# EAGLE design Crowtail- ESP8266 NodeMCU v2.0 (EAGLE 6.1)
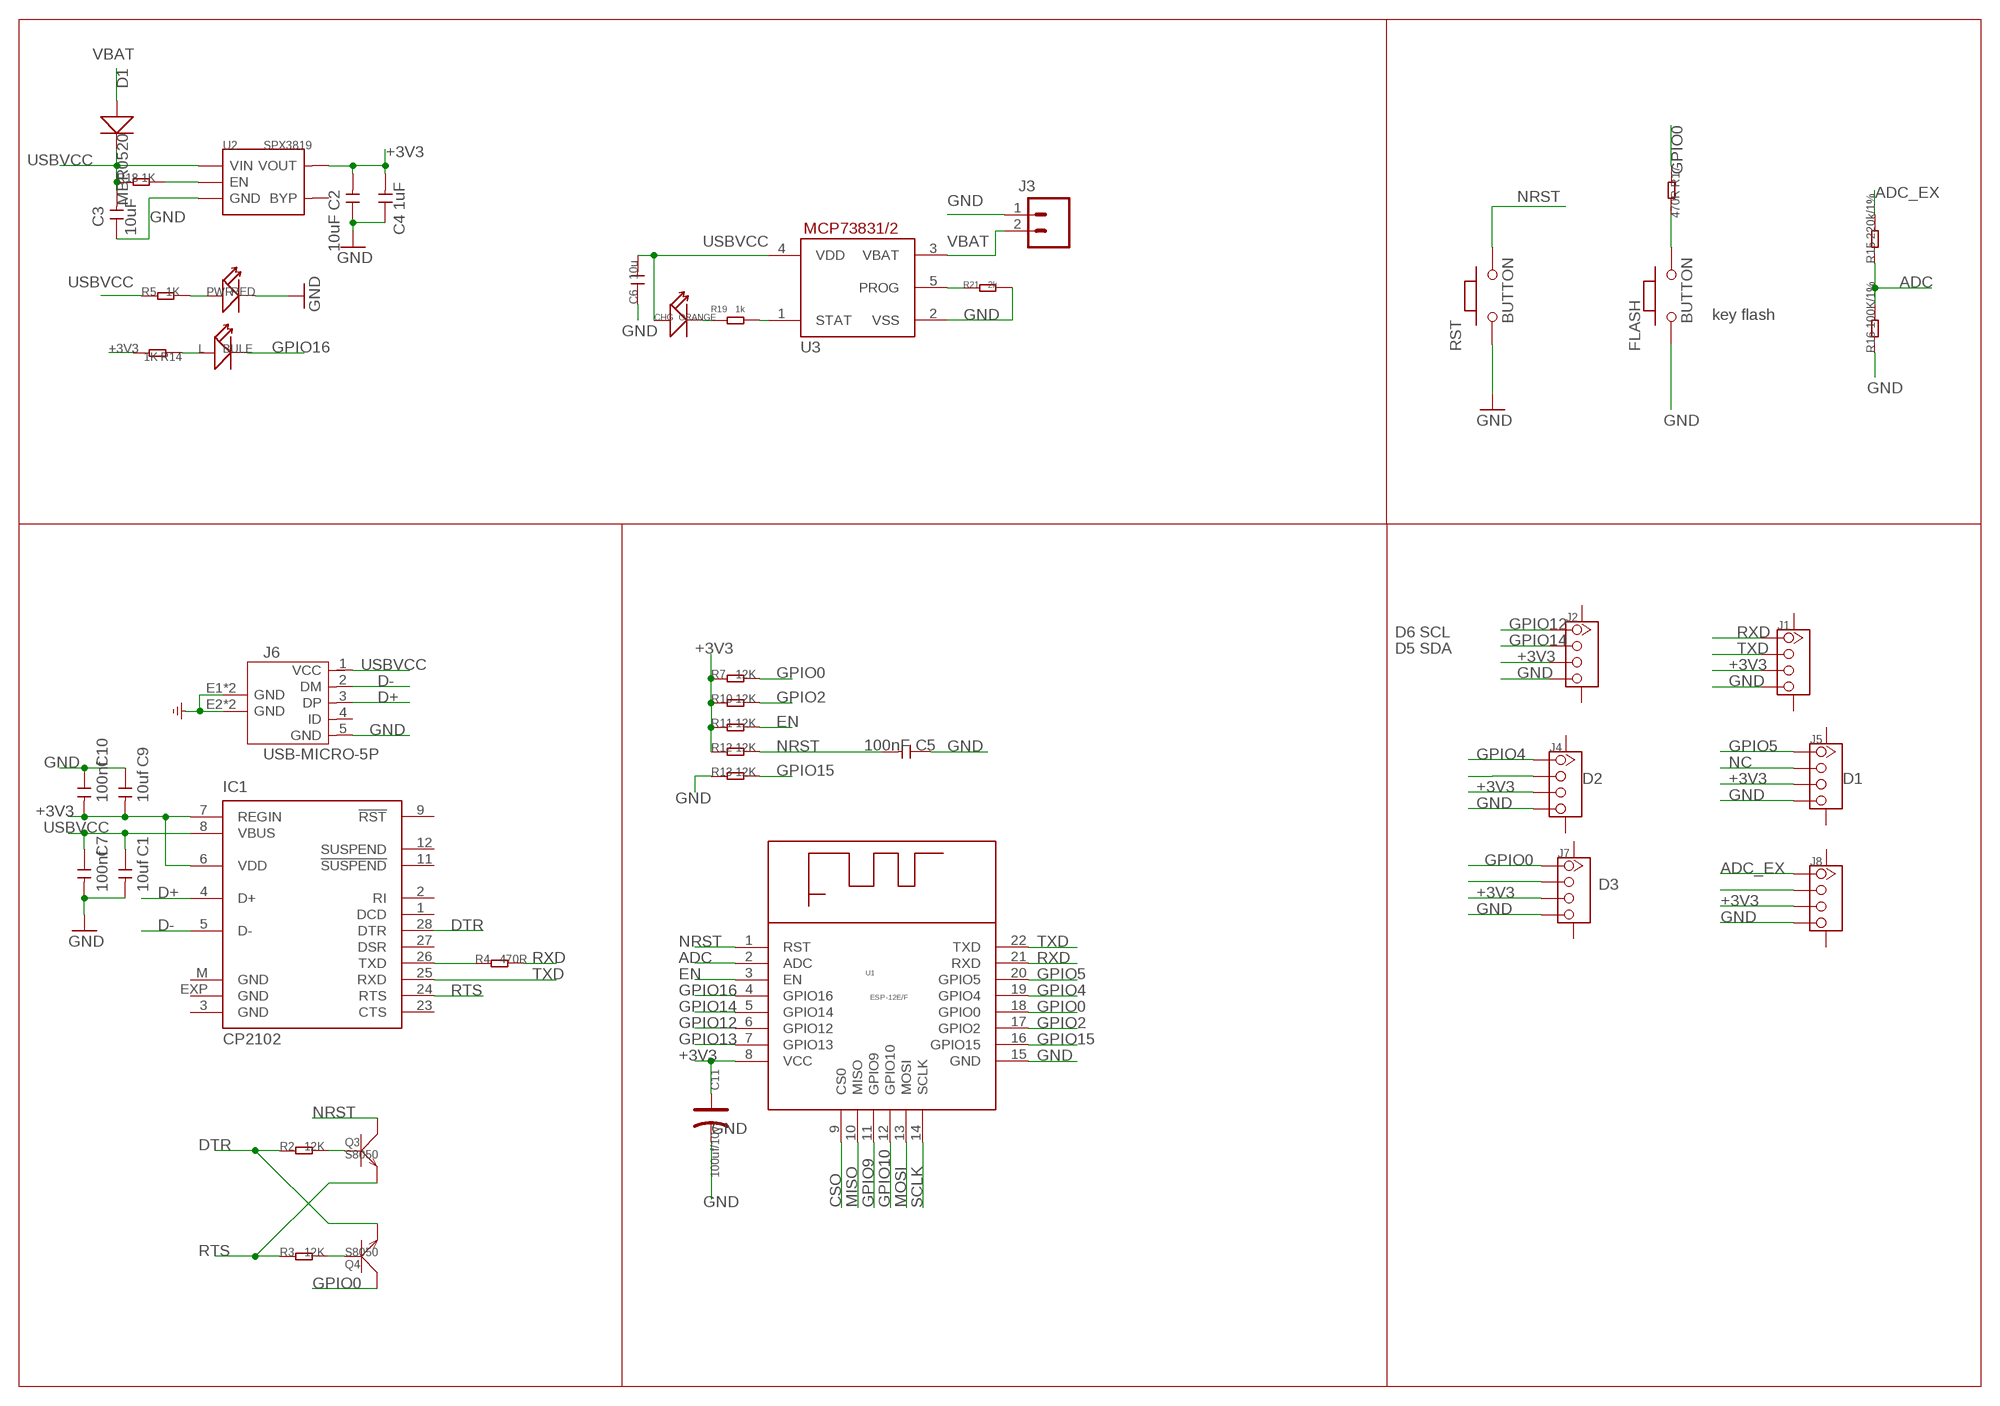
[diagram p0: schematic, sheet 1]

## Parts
C1  10uf  C-0603  [C0603]
C2  10uF  C-0603  [C0603]
C3  10uF  C-0603  [C0603]
C4  1uF  C-0603  [C0603]
C5  100nF  C-0603  [C0603]
C6  10u  C-0603  [C0603]
C7  100nf  C-0603  [C0603]
C9  10uf  C-0603  [C0603]
C10  100nf  C-0603  [C0603]
C11  100uf/10v  CAP-AVX-B  [AVX-B]
CHG  ORANGE  007-LED0603  [D0603]
D1  MBR0520  D'1206'  [SOD123]
FLASH  BUTTON  PB157  [157SW]
IC1  CP2102  [MLP28]
J1  TWIG-4P-2.0-SMD-FEMALE-REINFORCE'DD'  [4P-SMD-2.0]
J2  TWIG-4P-2.0-SMD-FEMALE-REINFORCE'DD'  [4P-SMD-2.0]
J3  M02-JST-2MM-SMT  [JST-2-SMD]
J4  TWIG-4P-2.0-SMD-FEMALE-REINFORCE'DD'  [4P-SMD-2.0]
J5  TWIG-4P-2.0-SMD-FEMALE-REINFORCE'DD'  [4P-SMD-2.0]
J6  USB-MICRO-5P  [MICRO-USB-5P]
J7  TWIG-4P-2.0-SMD-FEMALE-REINFORCE'DD'  [4P-SMD-2.0]
J8  TWIG-4P-2.0-SMD-FEMALE-REINFORCE'DD'  [4P-SMD-2.0]
L  BULE  LED'0603'  [LED-0603]
PWR  RED  LED'0603'  [LED-0603]
Q3  S8050  TRANSISTOR-NPN-SOT23  [SOT23]
Q4  S8050  TRANSISTOR-NPN-SOT23  [SOT23]
R2  12K  R-0603  [R0603]
R3  12K  R-0603  [R0603]
R4  470R  R-0603  [R0603]
R5  1K  R-0603  [R0603]
R7  12K  R-0603  [R0603]
R10  12K  R-0603  [R0603]
R11  12K  R-0603  [R0603]
R12  12K  R-0603  [R0603]
R13  12K  R-0603  [R0603]
R14  1K  R-0603  [R0603]
R15  220k/1%  R-0603  [R0603]
R16  100K/1%  R-0603  [R0603]
R17  470R  R-0603  [R0603]
R18  1K  R-0603  [R0603]
R19  1k  R-0603  [R0603]
R21  2k  R-0603  [R0603]
RST  BUTTON  PB157  [157SW]
U1  ESP-12E/F  [ESP-12E/F]
U2  SPX3819  [SOT23-5]
U3  MCP73831/OT  [SOT23-5L]

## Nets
+3V3: C2.2 C4.2 C9.2 C10.2 C11.+ IC1.6(VDD) IC1.7(REGIN) J1.3 J2.3 J4.3 J5.3 J7.3 J8.3 R7.1 R10.1 R11.1 R12.1 R14.2 U1.8(VCC) U2.5(VOUT)
ADC: R15.1 R16.2 U1.2(ADC)
ADC_EX: J8.1 R15.2
CSO: U1.9(CS0)
D+: IC1.4(D+) J6.3(DP)
D-: IC1.5(D-) J6.2(DM)
DTR: IC1.28(DTR) Q4.2(E) R2.1
EN: R11.2 U1.3(EN)
GND: C1.2 C2.1 C3.1 C4.1 C5.1 C6.1 C7.2 C9.1 C10.1 C11.- FLASH.1 J1.4 J2.4 J3.1 J4.4 J5.4 J6.5(GND) J6.E1(GND) J6.E2(GND) J6.P1(GND) J6.P2(GND) J7.4 J8.4 PWR.- R13.1 R16.1 R21.2 RST.1 U1.15(GND) U2.2(GND) U3.2(VSS)
GPIO0: J7.1 Q4.3(C) R7.2 R17.1 U1.18(GPIO0)
GPIO2: R10.2 U1.17(GPIO2)
GPIO4: J4.1 U1.19(GPIO4)
GPIO5: J5.1 U1.20(GPIO5)
GPIO9: U1.11(GPIO9)
GPIO10: U1.12(GPIO10)
GPIO12: J2.1 U1.6(GPIO12)
GPIO13: U1.7(GPIO13)
GPIO14: J2.2 U1.5(GPIO14)
GPIO15: R13.2 U1.16(GPIO15)
GPIO16: L.- U1.4(GPIO16)
M8TXD: IC1.26(TXD) R4.1
MISO: U1.10(MISO)
MOSI: U1.13(MOSI)
N$1: CHG.- R19.1
N$2: L.+ R14.1
N$3: PWR.+ R5.2
N$5: R18.2 U2.3(EN)
N$8: FLASH.2 R17.2
N$9: Q3.1(B) R2.2
N$10: Q4.1(B) R3.2
N$15: J4.2
N$20: R19.2 U3.1(STAT)
N$21: J7.2
N$25: J8.2
N$31: R21.1 U3.5(PROG)
NC: J5.2
NRST: C5.2 Q3.3(C) R12.2 RST.2 U1.1(RST)
RTS: IC1.24(RTS) Q3.2(E) R3.1
RXD: J1.1 R4.2 U1.21(RXD)
SCLK: U1.14(SCLK)
TXD: IC1.25(RXD) J1.2 U1.22(TXD)
USBVCC: C1.1 C3.2 C6.2 C7.1 CHG.+ D1.- IC1.8(VBUS) J6.1(VCC) R5.1 R18.1 U2.1(VIN) U3.4(VDD)
VBAT: D1.+ J3.2 U3.3(VBAT)
Unconnected: IC1.1(DCD) IC1.2(RI) IC1.9(!RST) IC1.11(!SUSPEND) IC1.12(SUSPEND) IC1.23(CTS) IC1.27(DSR) J1.SS1 J1.SS2 J2.SS1 J2.SS2 J4.SS1 J4.SS2 J5.SS1 J5.SS2 J6.4(ID) J7.SS1 J7.SS2 J8.SS1 J8.SS2 U2.4(BYP)

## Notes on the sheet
- 10k=100mA
- 5k=200mA
- 2k=500mA
- 1k=1000mA | key flash
- D6 SCL
- D5 SDA
- D2 | D1
- D3

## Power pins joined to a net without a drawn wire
GND: IC1.3(GND) IC1.EXP(GND) IC1.M(GND)

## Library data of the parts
C1-C7 C9 C10 = Discrete:C*: Ceramic Capacitors
C11 = Discrete:CAP*: Electrolytic Capacitors,Tantalum Capacitors and Super Capacitors
CHG = Discrete:007-LED*
D1 = Discrete:D*
FLASH RST = MySMD:PB157
IC1 = silabs:CP210*: Single-Chip USB to UART Bridge Source: www.silabs.com .. CP2101.pdf / cp2102.pdf; MF: FARNELL; MPN: CP2102-GM; OC_FARNELL: 9282130; OC_NEWARK: 30K5635
J1 J2 J4 J5 J7 J8 = Connector:TWIG-4P-2.0-SMD-FEMALE-REINFORCE
J3 = SparkFun:M02: Header 2
J6 = Connector:USB-MICRO-5P
L PWR = Discrete:LED*
Q3 Q4 = Discrete:TRANSISTOR-NPN*: NPN audion
R2-R5 R7 R10-R19 R21 = Discrete:R*
U1 = Discrete:ESP-12E/F
U2 = IC:SPX3819
U3 = adafruit:MCP73831: MCP73831/2 Miniature Single-Cell, Fully Integrated Li-Ion, Li-Polymer Charge Management Controllers. Nice and small simple lipoly charge controller, with adjustable current and status output (LED) http://www.ladyada.net/library/pcb/eaglelibrary.html

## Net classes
0 default: width 0.203 mm
1 power: width 0.61 mm, drill 0.61 mm, clearance 0.254 mm
2 gnd: width 0.305 mm, drill 0.559 mm, clearance 0.254 mm
3 usbvcc: width 0.508 mm, drill 0.61 mm, clearance 0.254 mm
4 aref: width 0.406 mm, drill 0.61 mm, clearance 0.254 mm

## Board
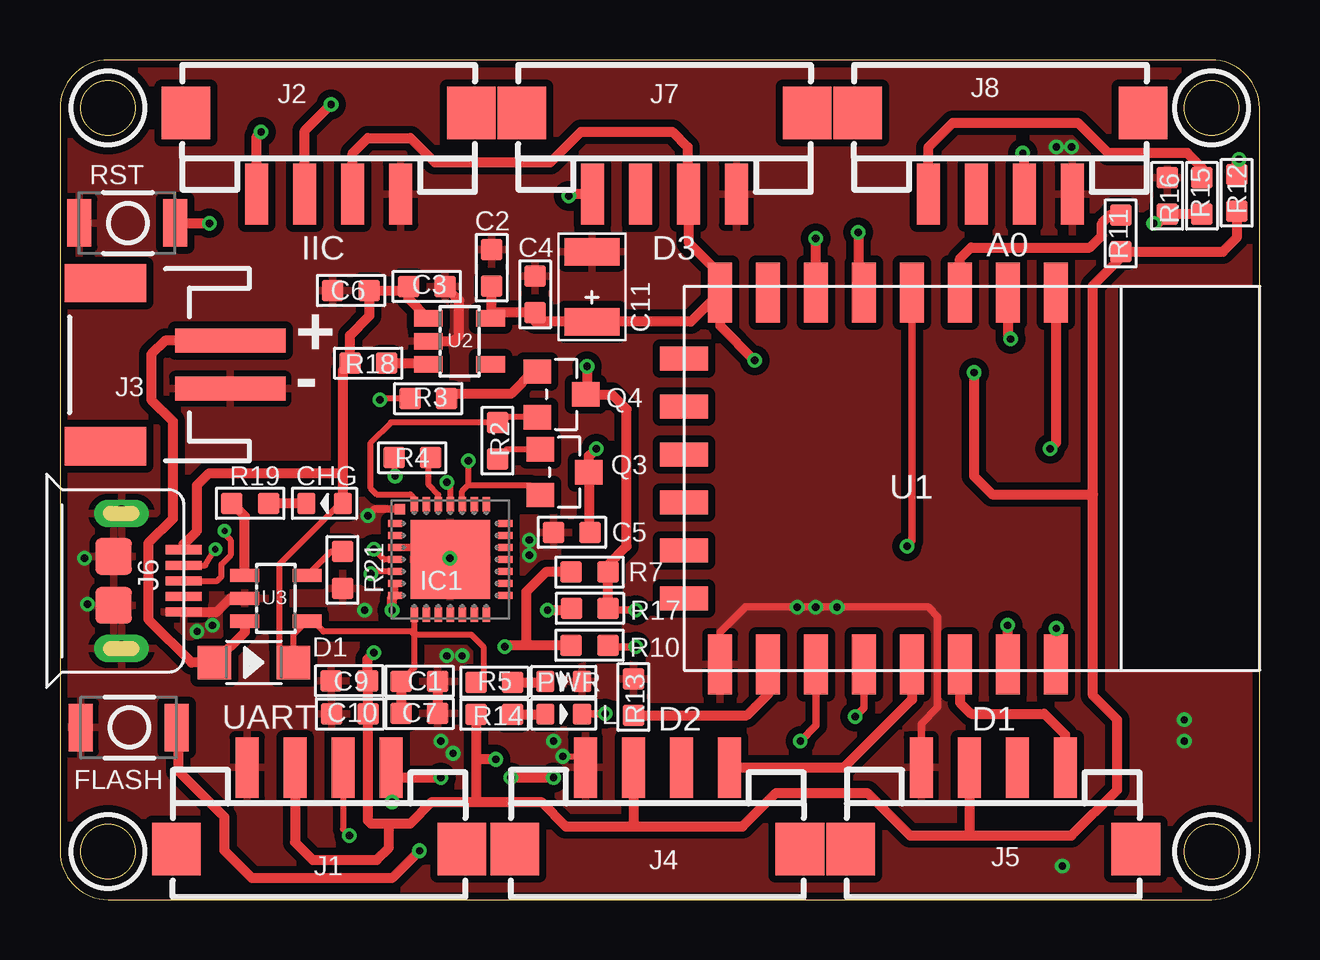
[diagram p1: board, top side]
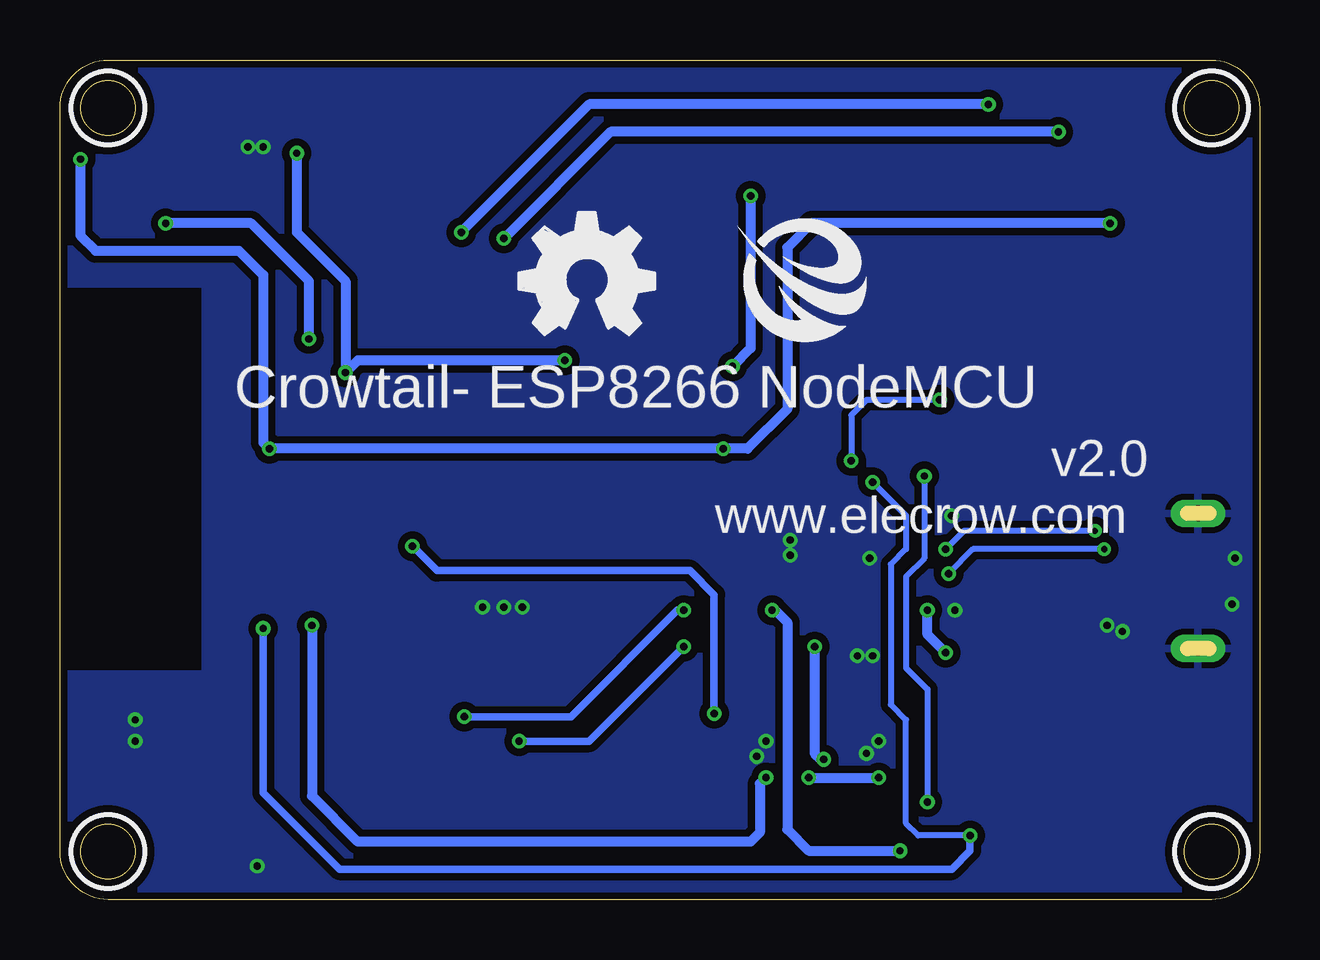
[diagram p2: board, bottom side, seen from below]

Size 50 x 35 mm. Coordinates in mm from the lower left corner, seen from the top.
Outline: 0,33 0,2 arc90 2,0 48,0 arc90 50,2 50,33 arc90 48,35 2,35 arc90 0,33
Outline: circle at 2,33 radius 1.14
Outline: circle at 48,33 radius 1.14
Outline: circle at 48,2 radius 1.14
Outline: circle at 2,2 radius 1.14
Copper layers (1*16): Top 0.035mm / dielectric 1.5mm / Bottom 0.035mm
Design rules: minimum track width 6mil, minimum drill 10mil, track to track 6mil, track to pad 6mil, pad to pad 6mil, via to via 6mil, smd to smd 0mil, copper to edge 10mil, drill to drill 10mil, minimum pad ring 10mil, minimum via ring 6mil, stop-mask expansion 2mil, vias tented up to drill 100mil, thermal gap 10mil
tRestrict: area 0.5,31.5 to 3.5,34.5; area 46.5,31.5 to 49.5,34.5; area 46.5,0.5 to 49.5,3.5; area 0.5,0.5 to 3.5,3.5
bRestrict: area 0.5,31.5 to 3.5,34.5; area 46.5,31.5 to 49.5,34.5; area 46.5,0.5 to 49.5,3.5; area 0.5,0.5 to 3.5,3.5

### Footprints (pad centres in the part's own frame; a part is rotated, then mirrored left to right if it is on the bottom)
C0603 = smd 0.889 x 0.889: 1 -0.762,0; 2 0.762,0
AVX-B = smd 1.143 x 2.286: + -1.46,0; - 1.46,0
D0603 = smd 0.762 x 0.889: + -0.762,0; - 0.762,0
SOD123 = smd 1.397 x 1.397: + -1.651,0; - 1.651,0
157SW = smd 1.016 x 1.981: 1 0,0; 2 4,0
MLP28 = smd 0.6 x 0.3: 1 -2.3,1.5; 2 -2.3,1; 3 -2.3,0.5; 4 -2.3,0; 5 -2.3,-0.5; 6 -2.3,-1; 7 -2.3,-1.5; 15 2.3,-1.5; 16 2.3,-1; 17 2.3,-0.5; 18 2.3,0; 19 2.3,0.5; 20 2.3,1; 21 2.3,1.5 | smd 0.3 x 0.6: 8 -1.5,-2.3; 9 -1,-2.3; 10 -0.5,-2.3; 11 0,-2.3; 12 0.5,-2.3; 13 1,-2.3; 14 1.5,-2.3; 22 1.5,2.3; 23 1,2.3; 24 0.5,2.3; 25 0,2.3; 26 -0.5,2.3; 27 -1,2.3; 28 -1.5,2.3 | smd 3.3 x 3.3: EXP 0,0 | smd 0.435 x 0.435: M -2.103,2.103
4P-SMD-2.0 = smd 0.965 x 2.54: 1 -3,0; 2 -1,0; 3 1,0; 4 3,0 | smd 2.032 x 2.184: SS1 -5.946,3.4; SS2 5.946,3.4
JST-2-SMD = smd 1 x 4.6: 1 -1,-3.7; 2 1,-3.7 | smd 1.6 x 3.4: NC1 -3.4,1.5; NC2 3.4,1.5
MICRO-USB-5P = smd 0.38 x 1.52: 1 -1.3,0; 2 -0.65,0; 3 0,0; 4 0.65,0; 5 1.3,0 | smd 1.524 x 1.524: E1 -1.016,-2.921; E2 1.016,-2.921 | drill 0.635 pad 1.143 long: P1 -2.819,-2.591; P2 2.819,-2.591
LED-0603 = smd 0.762 x 0.889: + -0.762,0; - 0.762,0
SOT23 = smd 1.016 x 1.143: 1 -0.95,-1.016; 2 0.95,-1.016; 3 0,1.016
R0603 = smd 0.889 x 0.889: 1 -0.762,0; 2 0.762,0
ESP-12E/F = smd 2.5 x 1: 1 0.25,15.5; 2 0.25,13.5; 3 0.25,11.5; 4 0.25,9.5; 5 0.25,7.5; 6 0.25,5.5; 7 0.25,3.5; 8 0.25,1.5; 15 15.75,1.5; 16 15.75,3.5; 17 15.75,5.5; 18 15.75,7.5; 19 15.75,9.5; 20 15.75,11.5; 21 15.75,13.5; 22 15.75,15.5 | smd 1 x 2: 9 3,0; 10 5,0; 11 7,0; 12 9,0; 13 11,0; 14 13,0
SOT23-5 = smd 0.69 x 1.2: 1 -0.95,-1.3; 2 0,-1.3; 3 0.95,-1.3; 4 0.95,1.3; 5 -0.95,1.3
SOT23-5L = smd 0.55 x 1.2: 1 -0.95,-1.3; 2 0,-1.3; 3 0.95,-1.3; 4 0.95,1.3; 5 -0.95,1.3

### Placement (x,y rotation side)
C1  14.99,9.1 0 top
C2  17.99,26.34 270 top
C3  15.29,25.56 180 top
C4  19.81,25.23 270 top
C5  21.34,15.31 0 top
C6  12.13,25.39 0 top
C7  14.98,7.75 0 top
C9  12.05,9.12 0 top
C10  12.09,7.73 0 top
C11  22.17,25.55 90 top
CHG  11.03,16.51 180 top
D1  8.09,9.88 0 top
FLASH  0.86,7.17 0 top
IC1  16.27,14.18 0 top
J1  10.8,5.5 180 top
J2  11.2,29.4 0 top
J3  3.4,22.3 90 top
J4  24.9,5.5 180 top
J5  38.9,5.5 180 top
J6  5.16,13.28 270 top
J7  25.2,29.4 0 top
J8  39.2,29.4 0 top
L  21,7.73 0 top
PWR  21,9.09 0 top
Q3  21.03,17.82 270 top
Q4  20.91,21.06 270 top
R2  18.23,19.13 270 top
R3  15.35,20.88 0 top
R4  14.68,18.42 180 top
R5  18.11,9.06 0 top
R7  22.07,13.65 0 top
R10  22.07,10.6 0 top
R11  44.21,27.77 90 top
R12  49.05,29.46 90 top
R13  23.9,8.44 270 top
R14  18.11,7.72 180 top
R15  47.6,29.34 90 top
R16  46.15,29.34 270 top
R17  22.09,12.14 180 top
R18  12.85,22.36 0 top
R19  7.93,16.52 180 top
R21  11.78,13.74 270 top
RST  0.8,28.2 0 top
U1  26.02,25.56 270 top
U2  16.65,23.27 270 top
U3  9,12.56 270 top
U$1  [ELECROW-NEW]  21.81,23.24 0 bottom
U$2  [OSHW_FILLX200_NOTEXT]  30.87,23.55 0 bottom

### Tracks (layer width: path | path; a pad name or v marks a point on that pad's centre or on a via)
+3V3  (via drill 0.3, 0.3 pad 0.25)
  Top 0.254: IC1.6 IC1.7
  Top 0.406: 13.72,3.17 12.95,3.17 12.83,3.3 12.83,7.73 C10.2 12.82,7.77 C9.2 12.82,10.02 v13.08,10.29 | 13.72,3.17 14.61,3.17 15.49,4.06 17.4,4.06 | 17.4,4.06 20.07,4.06 21.08,3.05 24,3.05 | 24,3.05 28.45,3.05 29.84,4.45 33.66,4.45 35.43,2.67 37.85,2.67 | 37.85,2.67 42.16,2.67 44.07,4.57 44.07,7.49 43.05,8.51 43.05,16.89 | 43.05,16.89 43.05,25.59 44.21,26.75 R11.1 48.47,27.01 49.05,27.58 R12.1 | J5.3 37.9,2.72 37.85,2.67 | J4.3 23.9,3.15 24,3.05 | R14.2 17.35,5.84 | 17.35,5.84 17.35,4.11 17.4,4.06 | J1.3 9.8,2.39 10.54,1.65 13.21,1.65 13.72,2.16 13.72,3.17 | v13.84,12.06 13.84,12.55 IC1.7 | R10.1 19.43,10.6 | 19.43,10.6 18.6,10.6 v18.54,10.54 | R7.1 20.25,13.65 19.43,12.83 19.43,10.6 | J8.3 40.2,31.05 v40.13,31.11 | v38.1,21.97 38.1,17.65 38.86,16.89 43.05,16.89 | U1.8 26.29,24.08 C11.+ 19.81,24.08 C4.2 18.2,24.47 U2.5 17.99,24.22 C2.2 | J2.3 12.2,31.12 12.83,31.75 14.61,31.75 15.62,30.73 20.45,30.73 21.72,32 25.53,32 26.16,31.37 26.16,29.44 J7.3 26.2,27.39 27.52,26.08 U1.8 | U1.8 27.52,23.92 v28.96,22.48 | v18.16,5.84 17.35,5.84
  Bottom 0.406: v13.08,10.29 13.84,11.05 v13.84,12.06 | v18.54,10.54 18.54,6.1 18.29,5.84 v18.16,5.84 | v40.13,31.11 40.13,27.81 38.1,25.78 v38.1,21.97 37.59,22.48 v28.96,22.48
ADC  (via drill 0.3 pad 0.25)
  Top 0.406: R15.1 R16.2 45.77,28.19 v45.59,28.19 | U1.2 39.52,23.48 v39.62,23.37
  Bottom 0.406: v39.62,23.37 39.62,25.78 42.04,28.19 v45.59,28.19
ADC_EX
  Top 0.406: R15.2 47.6,30.5 46.99,31.11 43.69,31.11 42.42,32.38 37.21,32.38 36.2,31.37 J8.1
D+  (via drill 0.25, 0.3)
  Top 0.254: J6.3 6.55,13.28 6.73,13.46 6.73,13.97 7.11,14.35 7.11,14.99 6.86,15.24 v6.86,15.37 | 13.21,14.48 v13.08,14.61 13.51,14.18 IC1.4
  Bottom 0.254: v13.08,14.61 12.32,15.37 v6.86,15.37
D-  (via drill 0.25, 0.3)
  Top 0.254: J6.2 6.06,13.93 v6.48,14.61 | IC1.5 13.04,13.68 v12.95,13.59
  Bottom 0.254: v6.48,14.61 11.94,14.61 v12.95,13.59
DTR
  Top 0.254: Q4.2 18.45,20.11 R2.1 13.8,19.89 12.95,19.05 12.95,17.14 13.21,16.89 14.61,16.89 14.77,16.73 IC1.28
EN
  Top 0.406: U1.3 37.52,26.72 37.97,27.18 42.93,27.18 43.43,27.69 43.43,28.19 43.77,28.53 R11.2
GND  (via drill 0.3)
  Top 0.254: v20.95,5.97 21.43,5.97 J4.4
  Top 0.305: J5.4 35.9,7.33 36.58,8 36.58,11.81 36.2,12.19 28.57,12.19 27.52,11.13 U1.15 | IC1.M 13.1,16.28 v12.83,16 | IC1.3 15.8,14.68 v16.26,14.22
  Top 0.406: C1.2 C7.2 | U2.2 16.41,23.27 16.64,23.5 16.64,24.97 C3.1 | J6.5 6.52,11.98 7.09,12.56 U3.2
  other vias: 12.7,12.06 19.56,14.35 19.56,14.99 15.88,6.6 16.38,6.1 16.13,10.16 16.76,10.16 20.57,6.6 5.71,11.18 1.14,12.32 1.02,14.22 6.35,11.43 41.53,31.37 42.16,31.37 46.86,7.49 41.78,1.4 46.86,6.6 30.73,12.19 31.5,12.19 32.38,12.19
  pour Top (isolate 0.305, rank 2): -0.13,35.43 50.29,35.43 50.29,25.65 43.94,25.65 43.94,9.4 50.04,9.4 50.04,0 -0.13,0
  pour Bottom (isolate 0.305, rank 2): -0.13,35.43 50.29,35.43 50.29,25.65 43.94,25.65 43.94,9.4 50.04,9.4 50.04,0 -0.13,0
GPIO0  (via drill 0.3, 0.3 pad 0.25)
  Top 0.305: U1.18 33.52,7.99 v33.15,7.62 | v24,12.06 22.92,12.06 R17.1
  Top 0.406: R17.1 22.85,13.63 R7.2 22.84,13.95 23.62,14.73 23.62,20.45 23.01,21.06 Q4.3 21.97,21.11 v21.97,22.23 | J7.1 21.27,29.4 v21.21,29.34
  Bottom 0.305: v33.15,7.62 28.7,7.62 24.26,12.06 v24,12.06
  Bottom 0.406: v21.21,29.34 21.21,22.99 v21.97,22.23
GPIO2  (via drill 0.3)
  Top 0.305: U1.17 31.52,7.26 v30.86,6.6 | v24,10.54 22.89,10.54 R10.2
  Bottom 0.305: v30.86,6.6 27.94,6.6 v24,10.54
GPIO4
  Top 0.406: J4.1 32.68,5.5 35.52,8.34 U1.19
GPIO5
  Top 0.406: U1.20 37.52,8.2 37.97,7.75 41.02,7.75 41.9,6.87 J5.1
GPIO12  (via drill 0.3 pad 0.25)
  Top 0.406: J2.1 8.2,31.82 v8.38,32 | v31.5,27.56 31.5,25.33 U1.6
  Bottom 0.406: v8.38,32 27.05,32 v31.5,27.56
GPIO14  (via drill 0.3 pad 0.25)
  Top 0.406: J2.2 10.2,32.04 v11.3,33.15 | v33.27,27.81 33.27,25.55 U1.5
  Bottom 0.406: v11.3,33.15 27.94,33.15 v33.27,27.81
GPIO15
  Top 0.406: U1.16 29.52,8.56 28.63,7.68 R13.2
GPIO16  (via drill 0.3)
  Top 0.305: L.- 22.72,7.73 v22.73,7.75 | 35.43,14.86 v35.31,14.73 35.52,14.94 U1.4
  Bottom 0.305: v22.73,7.75 22.73,12.7 23.75,13.72 34.29,13.72 v35.31,14.73
M8TXD
  Top 0.254: IC1.26 15.77,16.87 15.37,17.27 15.37,18.34 R4.1
N$1
  Top 0.406: CHG.- R19.1
N$2
  Top 0.406: R14.1 20.23,7.72 L.+
N$3
  Top 0.406: R5.2 20.23,9.06 PWR.+
N$5
  Top 0.406: R18.2 15.31,22.36 U2.3
N$8  (via drill 0.3, 0.3 pad 0.25)
  Top 0.406: FLASH.2 4.92,7.11 4.92,5.36 6.86,3.43 6.86,2.03 8,0.89 13.84,0.89 v14.99,2.03 | v20.32,12.06 21.25,12.06 R17.2
  Bottom 0.406: v14.99,2.03 18.8,2.03 19.68,2.92 19.68,11.56 20.19,12.06 v20.32,12.06
N$9
  Top 0.254: Q3.1 18.63,18.77 R2.2
N$10
  Top 0.406: Q4.1 19.72,22.01 18.8,21.08 16.31,21.08 R3.2
N$20
  Top 0.406: U3.1 7.7,15.98 R19.2
N$31
  Top 0.254: R21.1 11.29,14.5 U3.5
NRST  (via drill 0.3 pad 0.25)
  Top 0.406: C5.2 22.05,15.36 Q3.3 22.05,18.49 v22.35,18.8 | v41.27,18.8 41.53,19.05 41.53,25.29 U1.1 | R12.2 49.05,30.76 v49.15,30.86 | RST.2 v6.22,28.2 v6.22,28.19
  Bottom 0.406: v49.15,30.86 49.15,27.69 48.51,27.05 42.55,27.05 41.53,26.04 41.53,19.05 v41.27,18.8 v22.35,18.8 21.34,18.8 19.68,20.45 19.68,27.18 18.67,28.19 v6.22,28.19
RTS  (via drill 0.3)
  Top 0.254: IC1.24 16.77,17.02 17.02,17.27 | 17.02,17.27 19.61,17.27 Q3.2 | R3.1 13.39,20.88 v13.34,20.83 | v17.02,18.29 17.02,17.27
  Bottom 0.254: v13.34,20.83 16.38,20.83 17.02,20.19 v17.02,18.29
RXD  (via drill 0.3, 0.3 pad 0.25)
  Top 0.254: R4.2 13.92,17.7 v13.97,17.65 | v13.84,4.06 13.84,4.7 14.22,5.08
  Top 0.406: U1.21 39.52,11.41 v39.5,11.43 | v20.57,5.08 v18.8,5.08 | v15.88,5.08 14.22,5.08 J1.1
  Bottom 0.254: v13.97,17.65 13.97,14.22 14.73,13.46 14.73,9.65 13.84,8.76 v13.84,4.06
  Bottom 0.406: v20.57,5.08 20.83,4.83 20.83,2.79 21.21,2.41 37.59,2.41 39.5,4.32 v39.5,11.43 | v18.8,5.08 v15.88,5.08
TXD  (via drill 0.3)
  Top 0.254: J1.2 11.8,2.93 v12.06,2.67 | v16.13,17.4 16.26,17.27 16.26,16.49 IC1.25
  Top 0.406: U1.22 41.52,11.29 v41.53,11.3
  Bottom 0.254: v12.06,2.67 14.22,2.67 14.73,3.17 14.73,7.49 15.37,8.13 15.37,13.97 14.73,14.61 14.73,16 v16.13,17.4
  Bottom 0.305: v41.53,11.3 41.53,4.45 38.35,1.27 12.83,1.27 12.06,2.03 v12.06,2.67
USBVCC
  Top 0.254: IC1.8 14.77,11.05 | 14.77,11.05 14.77,9.65 C1.1 | 14.77,11.05 17.14,11.05 17.65,10.54 17.65,9.36 R5.1 | 14.77,11.05 14.64,11.18 10.98,11.18 10.55,11.61 U3.4 9.74,11.04 D1.- 9.14,10.47 9.14,13.97 11.69,16.51 CHG.+
  Top 0.406: C1.1 C7.1 | CHG.+ 11.79,17.91 | 11.79,17.91 11.79,22.07 R18.1 12.09,23.52 12.89,24.32 C6.2 14.37,25.39 C3.2 14.53,25.04 U2.1 | J6.1 5.16,14.81 5.71,15.37 5.71,17.27 6.22,17.78 11.66,17.78 11.79,17.91
VBAT
  Top 0.406: J3.2 4.38,23.3 3.81,22.73 3.81,20.83 4.7,19.94 4.7,15.88 3.68,14.86 3.68,11.68 5.49,9.88 D1.+ | D1.+ 6.43,10.09 | U3.3 7.7,11.14 D1.+

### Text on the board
tPlace: IIC | D3 | A0 | + | - | U1 | UART | D2 | D1
bNames: Crowtail- ESP8266 NodeMCU | v2.0 | www.elecrow.com
214bmp: D:/SmartProjects/Snc/a4_bn_logo2.bmp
